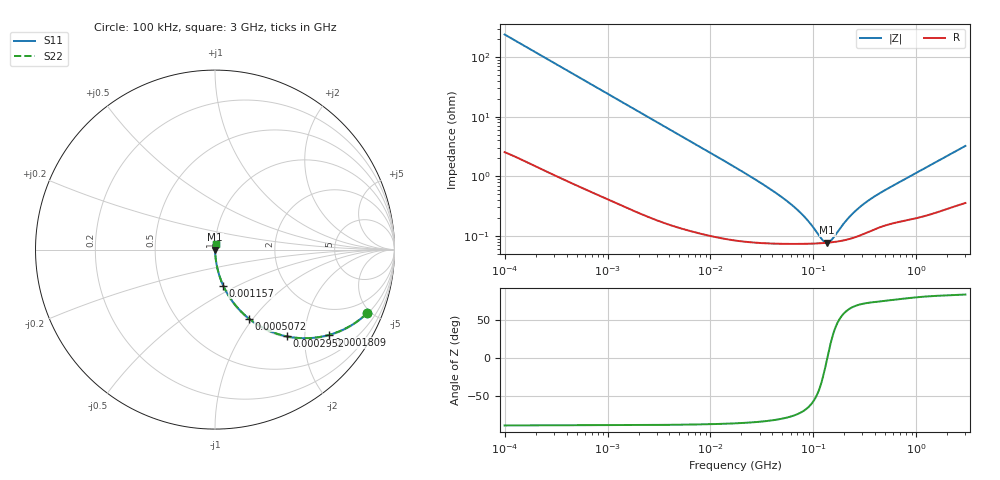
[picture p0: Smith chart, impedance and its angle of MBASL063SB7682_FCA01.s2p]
! MBASL063SB7682_FCA01  S-PARAMETER MODEL  ( Standard Model )
! Model Generated by TAIYO YUDEN Corporation (http://www.ty-top.com)
! Version 1.0
! TAIYO YUDEN Control No. 220601
! Copyright(c) 2020 TAIYO YUDEN CO.,LTD. All Rights Reserved.
! Product Description (link to TY-COMPAS)
! https://ds.yuden.co.jp/TYCOMPAS/or/detail?pn=MBASL063SB7682KFCA01&u=M
! Products Name : Multilayer Ceramic Capacitors
! Characteristics :
!  Capacitance : 6800 [pF] , Rated Voltage : 10 [V] , TCC : X7R
!  Case Size : 0.6 x 0.3 / 0.024 x 0.012 [mm/inch] , Thickness : 0.3 / 0.012 [mm/inch]
!  (Conditions: Temperature = 25 [degC] , DC Bias Voltage = 0 [V])
! External Node Assignments :
!  1  o---| |---o  2
! GND o---------o GND
! Frequency Range : 100kHz  -  3GHz  [ 401 STEP ]
# MHZ S RI R 50
! Freq[MHz].  S11 Real  S11 Imag  S21 Real  S21 Imag  S12 Real  S12 Imag  S22 Real  S22 Imag
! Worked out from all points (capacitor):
!   401 points, 100 kHz to 3 GHz, reference 50 ohm
!   read as one part in series: C = 6.66 nF near 105.3 kHz
!   lowest |Z| = 76.9 mohm at 136.1 MHz (marker M1)
!   series resonance near 136.7 MHz, so ESL is about 200 pH
!   S11 on the Smith chart (normalised r, x): 100 kHz: 1.05, -4.77; 180.9 kHz: 1.03, -2.65; 295.2 kHz: 1.02, -1.63; 507.2 kHz: 1.01, -0.95; 1.157 MHz: 1.01, -0.42; 3 GHz: 1.01, +0.06
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0.1  0.848 -0.3538  0.152 0.3538  0.152 0.3538  0.848 -0.3538
0.132776  0.7618 -0.4203  0.2382 0.4203  0.2382 0.4203  0.7618 -0.4203
0.180898  0.6356 -0.4753  0.3644 0.4753  0.3644 0.4753  0.6356 -0.4753
0.295187  0.4005 -0.4835  0.5995 0.4835  0.5995 0.4835  0.4005 -0.4835
0.507162  0.1886 -0.384  0.8114 0.384  0.8114 0.384  0.1886 -0.384
0.562235  0.1599 -0.3592  0.8401 0.3592  0.8401 0.3592  0.1599 -0.3592
0.786003  0.0907 -0.2793  0.9093 0.2793  0.9093 0.2793  0.0907 -0.2793
1.156955  0.0456 -0.2002  0.9544 0.2002  0.9544 0.2002  0.0456 -0.2002
3.161081  0.00775 -0.077  0.9923 0.077  0.9923 0.077  0.00775 -0.077
17.7727  0.00102 -0.0138  0.999 0.0138  0.999 0.0138  0.00102 -0.0138
34.73492  0.000797 -0.00673  0.9992 0.00673  0.9992 0.00673  0.000797 -0.00673
53.83243  0.000751 -0.00393  0.9992 0.00393  0.9992 0.00393  0.000751 -0.00393
75.25761  0.000741 -0.00232  0.9993 0.00232  0.9993 0.00232  0.000741 -0.00232
97.38194  0.000744 -0.00127  0.9993 0.00127  0.9993 0.00127  0.000744 -0.00127
122.8043  0.000758 -0.000393  0.9992 0.000393  0.9992 0.000393  0.000758 -0.000393
136.1397  0.000769 -1.38e-05  0.9992 1.38e-05  0.9992 1.38e-05  0.000769 -1.38e-05
150.9232  0.000783 0.000365  0.9992 -0.000365  0.9992 -0.000365  0.000783 0.000365
205.6221  0.000858 0.00154  0.9991 -0.00154  0.9991 -0.00154  0.000858 0.00154
266.0711  0.000983 0.0026  0.999 -0.0026  0.999 -0.0026  0.000983 0.0026
362.5028  0.00123 0.00401  0.9988 -0.00401  0.9988 -0.00401  0.00123 0.00401
547.5153  0.00161 0.00623  0.9984 -0.00623  0.9984 -0.00623  0.00161 0.00623
3000  0.00458 0.0319  0.9954 -0.0319  0.9954 -0.0319  0.00458 0.0319
